[IBIS Ver]   4.0
[File name]   mpc7410f_hcte.ibs
[File Rev]   0.3
[Date]   August 31, 2007
[Source]   File originated at Somerset. Created by Joshua Siegel.
[Notes]   This IBIS model is for the Rev1.4 MPC7410 360BGA HCTE package.
|   The driver and receiver models are characterized for
|   3.3V mode on the data bus and 1.8V mode on the L2
|   interface. The convention is mpc7410x_hcte.ibs, where x
|   is one of the configurations of data bus/L2 bus voltage
|   modes. Following is a table of the code for bus combinations:
|   IBIS model   Bus mode   L2 mode
|   mpc7410a_hcte.ibs   2.5V   2.5V
|   mpc7410b_hcte.ibs   2.5V   1.8V
|   mpc7410c_hcte.ibs   1.8V   2.5V
|   mpc7410d_hcte.ibs   1.8V   1.8V
|   mpc7410e_hcte.ibs   3.3V   2.5V
|   mpc7410f_hcte.ibs   3.3V   1.8V
|   You will see non-monotonicity in the pullup/pulldown data.
|   This accurately reflects the driver behavior and is not
|   a cause for concern.
|   Rev 03 Notes;
|   - Parse & check succeeded on all mpc7410x_hcte.ibs files.
[Disclaimer]   This information is for modeling purposes only and
|   is not guaranteed.
[Component]   MPC7410
[Manufacturer]  Freescale
[Package]
|   typ   min   max
R_pkg   0.165   0.014   0.300
L_pkg   5.917nH   0.606nH   11.000nH
C_pkg   1.127pF   0.099pF   2.090pF
[Pin]   signal_name   model_name  R_pin   L_pin   C_pin
 A02   TBEN   padio   0.271   8.10E-09   1.90E-12
 A03   EMODE_   padio   0.233   8.97E-09   1.59E-12
 A04   PLL_CFG0   padio   0.236   7.06E-09   1.64E-12
 A05   PLL_CFG1   padio   0.217   7.76E-09   1.49E-12
 A06   PLL_CFG2   padio   0.205   6.23E-09   1.47E-12
 A07   PLL_CFG3   padio   0.204   7.00E-09   1.30E-12
 A08   AVDD   POWER
 A09   TSIZ0   padio   0.167   5.93E-09   6.80E-13
 A10   TRST_   rcvr   0.151   5.63E-09   9.47E-13
 A11   TBST_   padio   0.147   4.56E-09   1.07E-12
 A12   SMI_   padio   0.147   5.17E-09   9.58E-13
 A13   A0   padio   0.134   5.32E-09   9.39E-13
 A14   L2D58   padiol2   0.162   6.37E-09   1.13E-12
 A15   L2D59   padiol2   0.179   7.00E-09   1.25E-12
 A16   L2D55   padiol2   0.197   7.71E-09   1.38E-12
 A17   L2D54   padiol2   0.215   8.41E-09   1.50E-12
 A18   L2D53   padiol2   0.234   9.12E-09   1.63E-12
 A19   L2VSEL   rcvr   0.247   8.49E-09   1.09E-12
 B01   GBL_   padio   0.229   8.80E-09   1.55E-12
 B02   QACK_   padio   0.215   8.22E-09   1.44E-12
 B03   SHD0_   padio   0.226   8.01E-09   1.53E-12
 B04   SHD1_   padio   0.191   7.32E-09   1.28E-12
 B05   HIT_   padio   0.174   6.76E-09   1.19E-12
 B06   HRESET_   padio   0.158   6.09E-09   1.06E-12
 B07   TDI   rcvr   0.174   6.23E-09   1.18E-12
 B08   CKSTOP_IN_   padio   0.158   4.84E-09   1.13E-12
 B09   TSIZ1   padio   0.141   5.20E-09   8.60E-13
 B10   TCK   rcvr   0.137   4.25E-09   9.90E-13
 B11   MCP_   padio   0.125   4.61E-09   7.59E-13
 B12   TT2   padio   0.118   4.20E-09   7.76E-13
 B13   A4   padio   0.114   4.54E-09   7.95E-13
 B14   L2D61   padiol2   0.147   5.36E-09   1.03E-12
 B15   L2DP7   padiol2   0.194   6.70E-09   1.24E-12
 B16   L2D56   padiol2   0.214   7.44E-09   9.15E-13
 B17   L2D52   padiol2   0.225   8.09E-09   1.57E-12
 B18   L2D51   padiol2   0.222   8.68E-09   1.55E-12
 B19   L2D50   padiol2   0.241   9.38E-09   1.68E-12
 C01   A3   padio   0.216   8.29E-09   1.46E-12
 C02   CI_   padio   0.227   8.85E-09   1.58E-12
 C03   WT_   padio   0.264   8.49E-09   1.89E-12
 C04   AP0   padio   0.195   6.96E-09   1.33E-12
 C05   AP1   padio   0.180   6.44E-09   1.23E-12
 C06   AP2   padio   0.175   6.27E-09   1.19E-12
 C07   AP3   padio   0.137   5.33E-09   9.26E-13
 C08   TMS   rcvr   0.118   4.56E-09   7.80E-13
 C09   TSIZ2   padio   0.114   4.34E-09   7.47E-13
 C10   TT0   padio   0.183   6.50E-09   1.19E-12
 C11   INT_   padio   0.103   3.64E-09   6.77E-13
 C12   TT3   padio   0.096   3.60E-09   5.86E-13
 C13   A6   padio   0.096   3.87E-09   6.73E-13
 C14   L2D62   padiol2   0.141   5.16E-09   9.86E-13
 C15   L2D60   padiol2   0.165   5.81E-09   1.16E-12
 C16   L2D57   padiol2   0.169   5.94E-09   7.04E-13
 C17   L2D49   padiol2   0.185   6.69E-09   1.29E-12
 C18   L2D48   padiol2   0.208   8.13E-09   1.45E-12
 C19   L2DP6   padiol2   0.227   8.84E-09   1.58E-12
 D01   DTI0   padio   0.206   7.90E-09   1.39E-12
 D02   A1   padio   0.171   6.60E-09   1.15E-12
 D03   RSRV_   padio   0.210   6.28E-09   1.45E-12
 D04   GND   POWER
 D05   OVDD   POWER
 D06   GND   POWER
 D07   CKSTP_OUT_   padio   0.098   3.83E-09   6.50E-13
 D08   OVDD   POWER
 D09   TDO   padio   0.096   3.71E-09   6.37E-13
 D10   GND   POWER
 D11   TT1   padio   0.083   2.65E-09   6.01E-13
 D12   OVDD   POWER
 D13   A8   padio   0.080   3.23E-09   5.56E-13
 D14   GND   POWER
 D15   L2OVDD   POWER
 D16   GND   POWER
 D17   L2D47   padiol2   0.190   6.55E-09   1.21E-12
 D18   L2D46   padiol2   0.194   7.59E-09   1.35E-12
 D19   L2D45   padiol2   0.210   8.19E-09   1.46E-12
 E01   A21   padio   0.164   6.43E-09   1.14E-12
 E02   A14   padio   0.200   7.18E-09   1.38E-12
 E03   CLK_OUT   padio   0.185   6.63E-09   1.27E-12
 E04   OVDD   POWER
 E05   A7   padio   0.115   4.42E-09   7.51E-13
 E06   OVDD   POWER
 E07   BR_   padio   0.159   5.63E-09   1.11E-12
 E08   GND   POWER
 E09   OVDD   POWER
 E10   SRESET_   padio   0.071   2.30E-09   5.32E-13
 E11   OVDD   POWER
 E12   GND   POWER
 E13   L2D63   padiol2   0.066   2.73E-09   4.64E-13
 E14   L2OVDD   POWER
 E15   L2D44   padiol2   0.129   4.73E-09   9.02E-13
 E16   L2OVDD   POWER
 E17   L2D43   padiol2   0.161   6.34E-09   1.13E-12
 E18   L2D42   padiol2   0.209   6.40E-09   1.52E-12
 E19   L2D41   padiol2   0.200   7.81E-09   1.39E-12
 F01   TA_   padio   0.185   6.88E-09   1.28E-12
 F02   A5   padio   0.154   5.72E-09   1.07E-12
 F03   A23   padio   0.177   6.40E-09   1.23E-12
 F04   GND   POWER
 F05   OVDD   POWER
 F06   GND   POWER
 F07   L2_TSTCLK   rcvr   0.108   3.94E-09   6.27E-13
 F08   L1_TSTCLK   rcvr   0.185   6.81E-09   1.28E-12
 F09   LSSD_MODE_   rcvr   0.211   6.73E-09   1.50E-12
 F10   GND   POWER
 F11   TT4   padio   0.094   3.22E-09   6.30E-13
 F12   A10   padio   0.038   1.42E-09   2.25E-13
 F13   L2D40   padiol2   0.101   3.19E-09   7.33E-13
 F14   GND   POWER
 F15   L2OVDD   POWER
 F16   GND   POWER
 F17   L2DP5   padiol2   0.149   5.86E-09   1.04E-12
 F18   L2D39   padiol2   0.174   6.82E-09   1.21E-12
 F19   L2D38   padiol2   0.193   7.55E-09   1.35E-12
 G01   DTI2   padio   0.247   8.91E-09   1.70E-12
 G02   A22   padio   0.143   4.38E-09   1.01E-12
 G03   A11   padio   0.120   3.70E-09   8.46E-13
 G04   A18   padio   0.114   3.48E-09   7.82E-13
 G05   A16   padio   0.071   2.70E-09   4.97E-13
 G06   A12   padio   0.057   2.15E-09   3.83E-13
 G07   A9   padio   0.018   8.27E-10   1.26E-13
 G08   VDD   POWER
 G09   GND   POWER
 G10   VDD   POWER
 G11   GND   POWER
 G12   VDD   POWER
 G13   L2D37   padiol2   0.155   5.12E-09   9.89E-13
 G14   L2D36   padiol2   0.105   3.35E-09   7.44E-13
 G15   L2D35   padiol2   0.125   3.89E-09   9.04E-13
 G16   L2D34   padiol2   0.116   4.26E-09   8.07E-13
 G17   L2ZZ   padiol2   0.178   5.94E-09   1.12E-12
 G18   L2A16   padiol2   0.159   5.77E-09   1.11E-12
 G19   L2D33   padiol2   0.175   6.86E-09   1.22E-12
 H01   BG   padio   0.246   8.26E-09   1.19E-12
 H02   A13   padio   0.141   4.93E-09   9.07E-13
 H03   A26   padio   0.108   3.41E-09   7.85E-13
 H04   OVDD   POWER
 H05   GND   POWER
 H06   DTI1   padio   0.275   9.26E-09   1.92E-12
 H07   A20   padio   0.026   9.71E-10   1.90E-13
 H08   GND   POWER
 H09   SYSCLK   padio   0.033   1.15E-09   2.20E-13
 H10   GND   POWER
 H11   A2   padio   0.014   6.06E-10   9.87E-14
 H12   GND   POWER
 H13   L2D32   padiol2   0.237   7.75E-09   1.58E-12
 H14   L2DP4   padiol2   0.088   2.80E-09   6.38E-13
 H15   GND   POWER
 H16   L2OVDD   POWER
 H17   L2A12   padiol2   0.148   5.31E-09   1.04E-12
 H18   L2A11   padiol2   0.146   5.75E-09   1.02E-12
 H19   L2A15   padiol2   0.167   6.55E-09   1.16E-12
 J01   TEA_   padio   0.244   8.71E-09   1.68E-12
 J02   A27   padio   0.136   4.98E-09   9.51E-13
 J03   QREQ_   padio   0.298   1.03E-08   2.07E-12
 J04   A19   padio   0.107   3.67E-09   6.49E-13
 J05   OVDD   POWER
 J06   A28   padio   0.277   8.92E-09   1.96E-12
 J07   A24   padio   0.089   3.04E-09   6.34E-13
 J08   VDD   POWER
 J09   GND   POWER
 J10   VDD   POWER
 J11   GND   POWER
 J12   VDD   POWER
 J13   L2A14   padiol2   0.055   1.84E-09   4.01E-13
 J14   L2A13   padiol2   0.075   2.42E-09   5.45E-13
 J15   L2OVDD   POWER
 J16   L2A10   padiol2   0.112   3.90E-09   6.97E-13
 J17   L2A9   padiol2   0.117   4.19E-09   8.32E-13
 J18   L2A8   padiol2   0.142   5.20E-09   9.94E-13
 J19   L2A7   padiol2   0.161   6.34E-09   1.12E-12
 K01   DBG_   padio   0.244   8.74E-09   1.69E-12
 K02   A30   padio   0.227   6.83E-09   1.59E-12
 K03   A29   padio   0.293   8.81E-09   2.09E-12
 K04   GND   POWER
 K05   DBB_   padio   0.167   5.62E-09   8.28E-13
 K06   GND   POWER
 K07   TS_   padio   0.194   5.78E-09   1.28E-12
 K08   GND   POWER
 K09   DRDY_   padio   0.055   1.82E-09   3.98E-13
 K10   GND   POWER
 K11   CHK_   rcvr   0.081   2.83E-09   5.80E-13
 K12   GND   POWER
 K13   L2OVDD   POWER
 K14   GND   POWER
 K15   L2A6   padiol2   0.077   2.47E-09   5.56E-13
 K16   GND   POWER
 K17   L2A5   padiol2   0.134   5.31E-09   9.36E-13
 K18   L2A4   padiol2   0.163   5.64E-09   1.04E-12
 K19   L2A17   padiol2   0.173   6.78E-09   1.21E-12
 L01   DP0   padio   0.160   5.36E-09   1.14E-12
 L02   A31   padio   0.193   7.57E-09   1.35E-12
 L03   A15   padio   0.175   6.66E-09   1.22E-12
 L04   A17   padio   0.156   5.93E-09   1.09E-12
 L05   OVDD   POWER
 L06   ARTRY_   padio   0.141   3.97E-09   1.08E-12
 L07   ABB_   padio   0.196   6.65E-09   1.34E-12
 L08   VDD   POWER
 L09   GND   POWER
 L10   VDD   POWER
 L11   GND   POWER
 L12   VDD   POWER
 L13   L2AVDD   POWER
 L14   L2SYNC_IN   padiol2   0.075   2.57E-09   4.56E-13
 L15   L2OVDD   POWER
 L16   L2CLK_OUTB   padiol2   0.084   3.40E-09   5.87E-13
 L17   L2A0   padiol2   0.125   4.52E-09   8.76E-13
 L18   L2A1   padiol2   0.136   5.40E-09   9.52E-13
 L19   L2A2   padiol2   0.177   6.94E-09   1.24E-12
 M01   DP4   padio   0.186   6.02E-09   1.24E-12
 M02   DP2   padio   0.162   5.51E-09   1.15E-12
 M03   A25   padio   0.180   6.82E-09   1.26E-12
 M04   OVDD   POWER
 M05   GND   POWER
 M06   D32   padio   0.249   9.47E-09   1.74E-12
 M07   D37   padio   0.047   1.64E-09   3.16E-13
 M08   GND   POWER
 M09   D8   padio   0.022   8.51E-10   1.61E-13
 M10   GND   POWER
 M11   D7   padio   0.105   3.70E-09   6.69E-13
 M12   GND   POWER
 M13   L2D30   padiol2   0.026   9.71E-10   1.90E-13
 M14   L2SYNC_OUT   padiol2   0.049   1.64E-09   3.53E-13
 M15   GND   POWER
 M16   L2OVDD   POWER
 M17   L2D29   padiol2   0.126   4.54E-09   8.87E-13
 M18   L2D31   padiol2   0.150   5.93E-09   1.05E-12
 M19   L2A3   padiol2   0.172   5.29E-09   1.24E-12
 N01   D59   padio   0.206   8.04E-09   1.44E-12
 N02   DP5   padio   0.166   5.67E-09   1.18E-12
 N03   AACK_   padio   0.299   9.81E-09   1.52E-12
 N04   D34   padio   0.167   6.07E-09   1.17E-12
 N05   D35   padio   0.130   4.47E-09   9.27E-13
 N06   D39   padio   0.204   7.81E-09   1.43E-12
 N07   D41   padio   0.053   1.79E-09   3.84E-13
 N08   VDD   POWER
 N09   GND   POWER
 N10   VDD   POWER
 N11   GND   POWER
 N12   VDD   POWER
 N13   L2D26   padiol2   0.025   9.24E-10   1.79E-13
 N14   L2D25   padiol2   0.044   1.73E-09   3.06E-13
 N15   L2CLK_OUTA   padiol2   0.099   3.50E-09   7.02E-13
 N16   L2WE_   padiol2   0.096   3.34E-09   5.94E-13
 N17   L2D28   padiol2   0.127   4.58E-09   8.88E-13
 N18   L2DP3   padiol2   0.149   5.86E-09   1.04E-12
 N19   L2D27   padiol2   0.169   6.62E-09   1.18E-12
 P01   D56   padio   0.221   8.64E-09   1.55E-12
 P02   DP1   padio   0.184   6.15E-09   1.22E-12
 P03   D33   padio   0.197   7.70E-09   1.37E-12
 P04   GND   POWER
 P05   OVDD   POWER
 P06   GND   POWER
 P07   D26   padio   0.070   2.86E-09   4.88E-13
 P08   D9   padio   0.052   2.01E-09   3.60E-13
 P09   D11   padio   0.053   1.77E-09   3.84E-13
 P10   GND   POWER
 P11   D42   padio   0.152   4.06E-09   1.26E-12
 P12   D45   padio   0.166   4.16E-09   1.50E-12
 P13   L2D24   padiol2   0.039   1.69E-09   2.74E-13
 P14   GND   POWER
 P15   L2OVDD   POWER
 P16   GND   POWER
 P17   L2CE_   padiol2   0.109   4.35E-09   7.61E-13
 P18   L2D23   padiol2   0.152   6.01E-09   1.06E-12
 P19   L2D22   padiol2   0.152   5.55E-09   1.06E-12
 R01   DP7   padio   0.224   7.80E-09   1.58E-12
 R02   D60   padio   0.228   8.91E-09   1.60E-12
 R03   D36   padio   0.241   8.44E-09   1.60E-12
 R04   OVDD   POWER
 R05   D31   padio   0.144   5.69E-09   1.01E-12
 R06   OVDD   POWER
 R07   D21   padio   0.078   3.18E-09   5.46E-13
 R08   GND   POWER
 R09   OVDD   POWER
 R10   D13   padio   0.123   3.84E-09   8.92E-13
 R11   OVDD   POWER
 R12   GND   POWER
 R13   L2D1   padiol2   0.182   6.99E-09   1.27E-12
 R14   L2OVDD   POWER
 R15   L2D21   padiol2   0.099   3.97E-09   6.91E-13
 R16   L2OVDD   POWER
 R17   L2D20   padiol2   0.137   5.42E-09   9.57E-13
 R18   L2D19   padiol2   0.157   5.72E-09   1.10E-12
 R19   L2D18   padiol2   0.171   6.19E-09   1.19E-12
 T01   D55   padio   0.266   9.55E-09   1.86E-12
 T02   D38   padio   0.240   9.37E-09   1.68E-12
 T03   DP6   padio   0.198   6.90E-09   1.29E-12
 T04   GND   POWER
 T05   OVDD   POWER
 T06   GND   POWER
 T07   D19   padio   0.116   4.26E-09   8.07E-13
 T08   OVDD   POWER
 T09   D3   padio   0.073   2.92E-09   4.66E-13
 T10   GND   POWER
 T11   D51   padio   0.210   6.20E-09   1.41E-12
 T12   OVDD   POWER
 T13   D46   padio   0.206   5.73E-09   1.57E-12
 T14   GND   POWER
 T15   L2OVDD   POWER
 T16   GND   POWER
 T17   L2D17   padiol2   0.163   6.42E-09   1.14E-12
 T18   L2D16   padiol2   0.180   7.06E-09   1.26E-12
 T19   L2DP2   padiol2   0.195   7.62E-09   1.36E-12
 U01   D58   padio   0.275   1.07E-08   1.92E-12
 U02   D40   padio   0.250   9.72E-09   1.74E-12
 U03   D62   padio   0.234   9.14E-09   1.64E-12
 U04   D30   padio   0.193   7.56E-09   1.35E-12
 U05   D24   padio   0.164   6.45E-09   1.15E-12
 U06   D22   padio   0.140   5.53E-09   9.77E-13
 U07   D20   padio   0.111   4.41E-09   7.73E-13
 U08   D17   padio   0.096   3.72E-09   6.25E-13
 U09   D5   padio   0.117   4.13E-09   7.14E-13
 U10   D6   padio   0.157   5.30E-09   1.05E-12
 U11   D52   padio   0.174   5.35E-09   1.26E-12
 U12   D44   padio   0.277   8.42E-09   2.01E-12
 U13   D48   padio   0.232   6.80E-09   1.57E-12
 U14   L2D0   padiol2   0.149   4.62E-09   1.08E-12
 U15   L2D5   padiol2   0.163   5.03E-09   1.18E-12
 U16   L2DP1   padiol2   0.174   5.37E-09   1.26E-12
 U17   L2D10   padiol2   0.188   5.77E-09   1.36E-12
 U18   L2D13   padiol2   0.197   7.73E-09   1.38E-12
 U19   L2D15   padiol2   0.217   6.62E-09   1.57E-12
 V01   D57   padio   0.281   1.01E-08   1.96E-12
 V02   DP3   padio   0.242   8.71E-09   1.69E-12
 V03   D61   padio   0.245   9.54E-09   1.71E-12
 V04   D28   padio   0.204   7.98E-09   1.43E-12
 V05   D27   padio   0.180   7.07E-09   1.26E-12
 V06   D16   padio   0.156   6.13E-09   1.09E-12
 V07   D15   padio   0.148   5.40E-09   1.03E-12
 V08   D54   padio   0.195   6.27E-09   1.40E-12
 V09   D18   padio   0.121   4.63E-09   7.88E-13
 V10   D49   padio   0.221   7.30E-09   1.50E-12
 V11   D2   padio   0.213   7.06E-09   1.42E-12
 V12   D53   padio   0.280   8.76E-09   1.85E-12
 V13   D43   padio   0.261   6.99E-09   1.91E-12
 V14   L2DP0   padiol2   0.167   6.07E-09   1.17E-12
 V15   L2D4   padiol2   0.177   6.41E-09   1.23E-12
 V16   L2D7   padiol2   0.200   7.24E-09   1.40E-12
 V17   L2D9   padiol2   0.201   7.87E-09   1.40E-12
 V18   L2D12   padiol2   0.224   8.08E-09   1.57E-12
 V19   L2D14   padiol2   0.230   8.95E-09   1.60E-12
 W01   BVSEL   rcvr   0.282   1.10E-08   1.97E-12
 W02   D63   padio   0.280   1.09E-08   1.96E-12
 W03   D29   padio   0.239   9.32E-09   1.67E-12
 W04   D25   padio   0.220   8.60E-09   1.54E-12
 W05   D23   padio   0.197   7.73E-09   1.38E-12
 W06   D14   padio   0.167   6.55E-09   1.16E-12
 W07   D10   padio   0.148   5.84E-09   1.03E-12
 W08   D50   padio   0.215   7.48E-09   1.40E-12
 W09   D12   padio   0.149   5.44E-09   1.04E-12
 W10   D4   padio   0.149   5.43E-09   1.04E-12
 W11   D1   padio   0.166   5.67E-09   1.18E-12
 W12   D0   padio   0.214   7.08E-09   1.53E-12
 W13   D47   padio   0.284   9.68E-09   1.21E-12
 W14   L2D2   padiol2   0.189   6.85E-09   1.32E-12
 W15   L2D3   padiol2   0.191   7.47E-09   1.33E-12
 W16   L2D6   padiol2   0.209   7.54E-09   1.46E-12
 W17   L2D8   padiol2   0.230   8.26E-09   1.60E-12
 W18   L2D11   padiol2   0.247   8.86E-09   1.72E-12
 W19   L2A18   padiol2   0.300   1.03E-08   1.95E-12
| Models and submodels in the file (3): padio (I/O), rcvr (Input), padiol2 (I/O)
